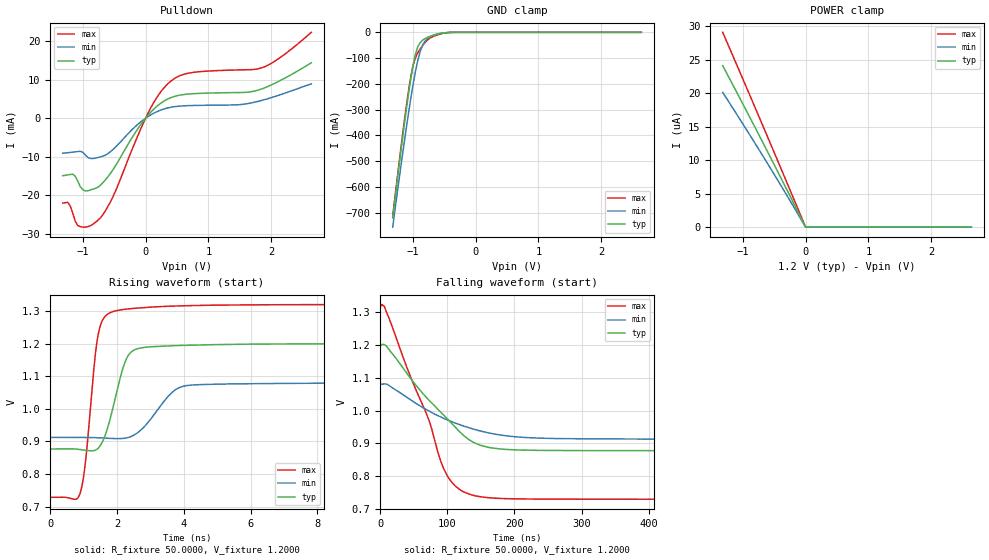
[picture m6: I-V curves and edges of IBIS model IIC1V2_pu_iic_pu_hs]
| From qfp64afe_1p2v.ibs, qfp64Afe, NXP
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[Model] IIC1V2_pu_iic_pu_hs
|   Model IIC1V2_pu_iic_pu_hs
| This model was characterised for following simulation conditions:
| External (pad) voltage:
|   - Typ: 1.2V,   - Min: 1.08V,   - Max: 1.32V
| Library cells for typ/min/max conditions are connected as defined below:
|  IO - External Pad
|  A - Core Input
|  EN - Output Buffer Enable
|  BOOST - vdde
|  ECS - vdd
|  EGP - gnd
|  ENZI - vdd
|  EPD - gnd
|  EPUN - gnd
|  SSEL - vdd
|  ZI - NC
|  ZIF - NC
|  gnd - gnd
|  gnde - gnde
|  vdd - vdd
|  vdde - vdde
| All other pins connected to ground
Model_type I/O_open_drain
Polarity   Non-Inverting
Enable   Active-Low
Vinl =   0.5400V
Vinh =   1.2600V
Vmeas =  0.9000V
Cref =   0.0F
Rref =   1.0000k
Vref =   1.2000V
C_comp   3.6132pF   3.4729pF   3.7394pF
|C_comp_pullup   0.9302pF   0.8892pF   0.9447pF
|C_comp_pulldown   2.3308pF   2.4848pF   2.1849pF
[Model Spec]
| variable   typ   min   max
Vinh   0.3600V   0.3240V   0.3960V
Vinl   0.8400V   0.7560V   0.9240V
Vmeas   0.6000V   0.5400V   0.6600V
Vref   1.2000V   1.0800V   1.3200V
Cref   0.0F   0.0F   0.0F
Rref   1.0000k   1.0000k   1.0000k
[Temperature Range]   25.0000   0.1250k   -40.0000
[Voltage Range]   1.2000V   1.0800V   1.3200V
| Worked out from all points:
|   slope of the pulldown table from 0 to 0.18 V, typ, clamps not added: 58.3 ohm
|   GND clamp passes 1 mA (typ) near -0.45 V on its own axis
|   rising waveform, R_fixture 50.0000, V_fixture 1.2000: 20-80 % time 494ps typ, 787ps min, 328ps max; typ from 0.877 V to 1.2 V
|   falling waveform, R_fixture 50.0000, V_fixture 1.2000: 20-80 % time 83.4ns typ, 99ns min, 62.7ns max; typ from 1.2 V to 0.877 V
[Pulldown]
|Voltage   I(typ)   I(min)   I(max)
-1.32V    -14.96mA   -9.099mA   -22.09mA
-1.24V    -14.75mA   -8.982mA   -21.89mA
-1.16V    -14.56mA   -8.83mA    -24.7mA
-1.04V    -17.82mA   -8.609mA   -28.21mA
-920mV    -18.88mA   -10.21mA   -28.21mA
-720mV    -17.44mA   -10.07mA   -25.94mA
-520mV    -13.41mA   -8.157mA   -20.44mA
80mV      1.521mA    840uA      2.628mA
440mV     5.569mA    2.951mA    10.1mA
760mV     6.377mA    3.307mA    11.92mA
1.84V     7.555mA    4.581mA    13.06mA
2.64V     14.41mA    8.944mA    22.34mA
[GND_clamp]
|Voltage   I(typ)   I(min)   I(max)
-1.32V    -720.7mA   -756.5mA   -713.8mA
-1.12V    -330.9mA   -399.5mA   -316.8mA
-1.04V    -192.5mA   -269.2mA   -184.5mA
-1V       -133.6mA   -209.3mA   -133.5mA
-960mV    -86.76mA   -154.8mA   -99.49mA
-920mV    -55.71mA   -108.2mA   -79.05mA
-880mV    -39.04mA   -72.36mA   -63.74mA
-840mV    -29.93mA   -48.01mA   -50.29mA
-760mV    -18.95mA   -23.41mA   -28.35mA
-640mV    -9.243mA   -8.645mA   -12.76mA
-400mV    -357.8uA   -419.3uA   -472.1uA
2.64V     0A         0A         0A
[POWER_clamp]
|Voltage   I(typ)   I(min)   I(max)
-1.32V    24.09uA    20.1uA     29.06uA
-640mV    11.88uA    10.01uA    14.23uA
0V        86.89pA    4.342nA    7.851pA
2.64V     0A         0A         0A
[Ramp]
| variable   typ   min   max
dV/dt_r  0.1939/0.4940n   0.1006/0.7872n   0.3549/0.3280n
dV/dt_f  0.1938/83.3502n   0.1006/98.9866n   0.3549/62.6840n
R_load = 50.0000
[Rising Waveform]
R_fixture= 50.0000
V_fixture= 1.2000
V_fixture_min= 1.0800
V_fixture_max= 1.3200
|time   V(typ)   V(min)   V(max)
0s        876.9mV    912.3mV    728.5mV
903.9ps   875.1mV    912.6mV    744.4mV
1.064ns   872.9mV    912.5mV    845.7mV
1.398ns   876mV      911.4mV    1.206V
1.674ns   927.6mV    910mV      1.287V
2.165ns   1.121V     909.1mV    1.304V
2.468ns   1.178V     917.3mV    1.308V
3.864ns   1.194V     1.065V     1.316V
6.251ns   1.198V     1.077V     1.319V
1us       1.2V       1.08V      1.32V
[Falling Waveform]
R_fixture= 50.0000
V_fixture= 1.2000
V_fixture_min= 1.0800
V_fixture_max= 1.3200
|time   V(typ)   V(min)   V(max)
0s        1.2V       1.08V      1.32V
6.494ns   1.2V       1.081V     1.316V
39.37ns   1.114V     1.041V     1.133V
72.8ns    1.031V     998mV      969.1mV
95.06ns   984.7mV    975.5mV    819.9mV
112.2ns   948.1mV    961.3mV    768.4mV
135.1ns   907.2mV    945.4mV    742.7mV
174.2ns   883.4mV    926.7mV    731.8mV
265ns     877.7mV    914.2mV    729.1mV
1us       877mV      912.4mV    728.6mV
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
